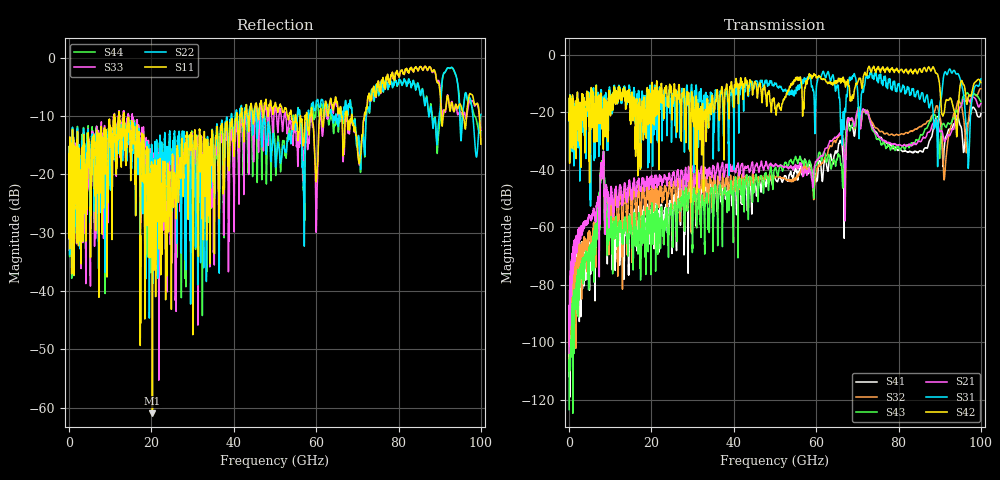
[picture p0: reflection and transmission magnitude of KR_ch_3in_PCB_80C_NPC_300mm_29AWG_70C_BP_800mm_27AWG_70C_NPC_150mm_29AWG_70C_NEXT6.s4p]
# Hz S RI R 45
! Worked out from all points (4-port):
!   4000 points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, 25 MHz to 100 GHz, reference 45 ohm
!   strongest paths, dB at 25 MHz, 25.02 GHz, 50.02 GHz, 75.03 GHz, 100 GHz:
!     S42: -20.7, -20.7, -18.8, -4.2, -9.7
!     S31: -20.7, -15.6, -10.1, -9.3, -8.4
!     S21: -103.8, -43.0, -38.3, -28.3, -17.0
!     S43: -123.5, -60.1, -39.5, -29.5, -16.4
!     S32: -108.5, -51.7, -42.9, -25.9, -11.9
!     S41: -112.1, -68.8, -43.0, -28.0, -20.5
!   lowest |S11| = -61.0 dB at 20.25 GHz (marker M1), VSWR 1.00, Z = 45 - j0.0803 ohm
!   |S11| at or under -10 dB: start of sweep to 10.95 GHz; 13.32 GHz to 40.64 GHz (27.31 GHz wide, 101 % of centre); 68.72 GHz to 71.7 GHz (2.978 GHz wide, 4.24 % of centre)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
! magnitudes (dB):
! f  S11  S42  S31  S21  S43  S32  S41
! 25 MHz  -16.5  -20.7  -20.7  -103.8  -123.5  -108.5  -112.1
! 8.025 GHz  -28.5  -24.8  -24.7  -41.8  -38.7  -40.3  -39.0
! 20.25 GHz  -61.0  -11.9  -26.2  -46.1  -56.1  -50.8  -56.7
! 72.05 GHz  -9.4  -7.1  -7.8  -20.3  -20.6  -20.4  -20.0
! 91.25 GHz  -9.0  -18.2  -6.1  -30.3  -24.8  -41.5  -30.2
! 96.85 GHz  -7.7  -15.3  -36.1  -15.2  -13.4  -24.4  -23.8
! 100 GHz  -14.8  -9.7  -8.4  -17.0  -16.4  -11.9  -20.5
